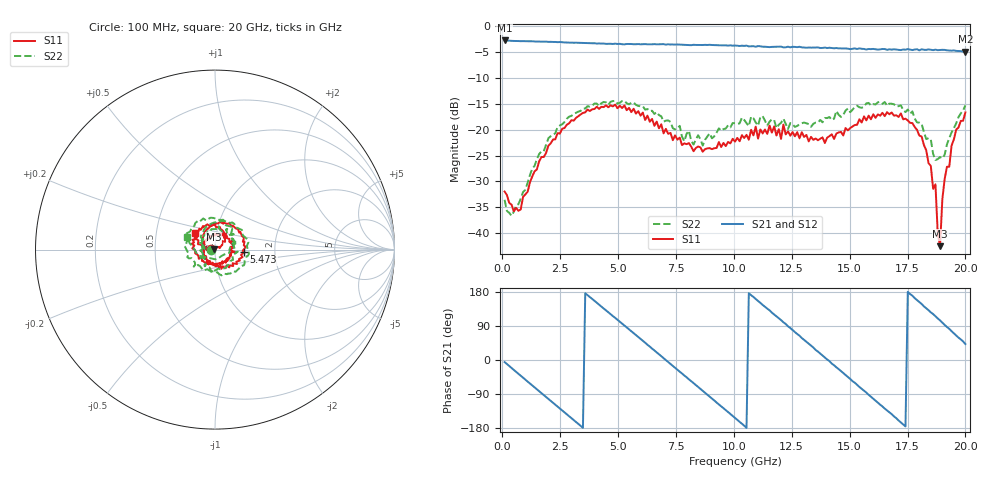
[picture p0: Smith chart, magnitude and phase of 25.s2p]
!Agilent Technologies,N5230C,MY49001569,A.09.33.09
!Agilent N5230C: A.09.33.09
!Date: Tuesday, July 21, 2015 09:58:53
!Correction: S11(Full 2 Port(1,2))
!S21(Full 2 Port(1,2))
!S12(Full 2 Port(1,2))
!S22(Full 2 Port(1,2))
!S2P File: Measurements: S11, S21, S12, S22:
# Hz S  dB  R 50
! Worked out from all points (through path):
!   201 points, 100 MHz to 20 GHz, reference 50 ohm
!   highest |S21| = -2.72 dB at 100 MHz (marker M1); lowest = -4.9 dB at 20 GHz (marker M2)
!   group delay of S21, straight-line fit = 143 ps
!   lowest |S11| = -42.6 dB at 18.91 GHz (marker M3), VSWR 1.02, Z = 49.3 + j0.148 ohm
!   |S11| at or under -10 dB: start of sweep to end of sweep
!   |S22| runs from -36.7 to -14.4 dB; largest |S21 - S12| = 0.019
!   S11 on the Smith chart (normalised r, x): 100 MHz: 0.95, +0.01; 5.473 GHz: 1.39, -0.04; 20 GHz: 0.78, +0.15
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1e8  -31.98 173.6  -2.72 -5.5  -2.71 -5.5  -33.58 -179.7
7.965e8  -35.44 -166.9  -2.86 -41.4  -2.84 -41.5  -33.36 -165.5
1.7915e9  -25.28 167.9  -2.96 -92.6  -2.95 -92.6  -24.17 167.4
3.483e9  -16.75 90.2  -3.20 -178.8  -3.23 -179.0  -15.89 83.8
4.5775e9  -15.66 35.0  -3.37 125.9  -3.34 126.0  -15.19 27.4
5.473e9  -15.78 -5.2  -3.40 80.8  -3.41 81.1  -15.08 -20.2
6.7665e9  -19.74 -65.0  -3.46 15.2  -3.46 15.1  -17.17 -80.2
8.5575e9  -23.43 -157.6  -3.61 -76.2  -3.57 -76.4  -21.88 -177.1
1.005e10  -22.30 96.9  -3.70 -152.9  -3.71 -153.0  -18.75 99.2
1.09455e10  -19.41 54.6  -3.94 161.0  -3.78 160.6  -18.60 56.0
1.19405e10  -19.90 5.4  -3.94 110.2  -3.96 109.4  -19.04 1.1
1.3433e10  -21.97 -68.6  -4.11 33.0  -4.13 32.5  -18.86 -87.6
1.4428e10  -20.76 -120.9  -4.18 -19.4  -4.22 -19.0  -16.37 -141.4
1.5423e10  -17.98 177.2  -4.26 -71.2  -4.35 -70.9  -15.67 170.1
1.67165e10  -17.01 116.4  -4.43 -138.4  -4.40 -138.0  -14.95 98.2
1.81095e10  -21.31 50.0  -4.43 147.9  -4.52 147.8  -18.85 21.7
1.87065e10  -30.58 32.6  -4.50 115.3  -4.51 115.2  -25.87 -44.0
1.8806e10  -40.05 61.2  -4.60 109.6  -4.58 109.1  -25.69 -69.8
1.89055e10  -42.55 168.4  -4.56 104.6  -4.58 103.6  -25.30 -88.2
1.9005e10  -33.45 -179.2  -4.53 98.5  -4.57 97.8  -25.55 -97.2
1.9204e10  -27.18 -177.1  -4.63 87.0  -4.57 87.2  -22.84 -146.5
2e10  -16.66 140.2  -4.90 42.2  -4.84 42.7  -15.28 156.7
